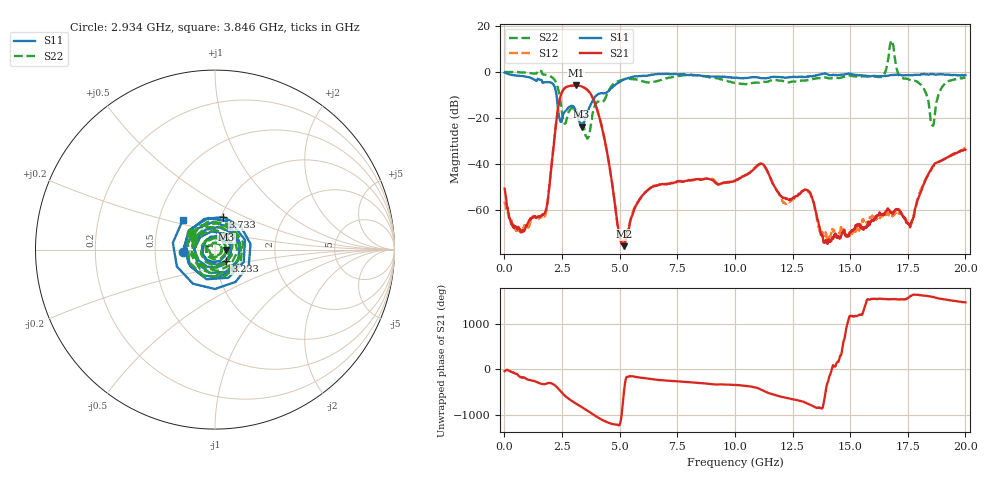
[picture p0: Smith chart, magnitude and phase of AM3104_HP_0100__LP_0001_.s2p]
!Created with skrf (http://scikit-rf.org).
# Hz S RI R 50.0
!freq ReS11 ImS11 ReS21 ImS21 ReS12 ImS12 ReS22 ImS22
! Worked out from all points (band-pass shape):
!   1601 points, 10 MHz to 20 GHz, reference 50 ohm
!   highest |S21| = -5.89 dB at 3.108 GHz (marker M1); lowest = -75.9 dB at 5.207 GHz (marker M2)
!   |S21| within 3 dB of the highest: 2.494 GHz to 3.696 GHz (1.201 GHz wide, 38.8 % of centre)
!   lowest |S11| = -23.9 dB at 3.346 GHz (marker M3), VSWR 1.14, Z = 56.8 - j0.0804 ohm
!   |S11| at or under -10 dB: 2.26 GHz to 4.026 GHz (1.766 GHz wide, 56.2 % of centre)
!   |S22| runs from -29.2 to 13.7 dB; largest |S21 - S12| = 0.028
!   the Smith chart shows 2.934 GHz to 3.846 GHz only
!   S11 on the Smith chart (normalised r, x): 2.934 GHz: 0.69, -0.02; 3.233 GHz: 1.11, -0.15; 3.733 GHz: 1.02, +0.38; 3.846 GHz: 0.66, +0.23
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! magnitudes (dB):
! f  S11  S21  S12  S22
! 10 MHz  -0.3  -50.8  -56.5  0.0
! 747.1 MHz  -1.8  -69.9  -69.1  -0.3
! 1.722 GHz  -4.6  -62.0  -62.8  -1.2
! 2.396 GHz  -20.5  -12.2  -12.2  -10.6
! 2.934 GHz  -14.8  -6.0  -6.0  -15.8
! 3.108 GHz  -17.0  -5.9  -5.9  -17.0
! 3.233 GHz  -21.2  -6.0  -6.1  -18.7
! 3.346 GHz  -23.9  -6.3  -6.4  -20.9
! 3.733 GHz  -14.6  -9.4  -9.5  -24.1
! 3.846 GHz  -12.3  -11.5  -11.5  -17.4
! 5.207 GHz  -3.2  -75.9  -74.4  -3.2
! 6.682 GHz  -0.9  -49.2  -49.3  -3.9
! 10.01 GHz  -2.6  -47.6  -47.4  -4.8
! 11.15 GHz  -2.8  -40.0  -40.2  -4.5
! 12.14 GHz  -2.5  -54.8  -56.9  -4.1
! 13.34 GHz  -2.0  -54.5  -54.7  -3.3
! 13.94 GHz  -0.8  -73.2  -70.3  -2.5
! 16.68 GHz  -1.5  -60.3  -62.5  7.2
! 17.63 GHz  -1.4  -66.7  -66.3  -3.5
! 18.56 GHz  -0.9  -41.4  -41.8  -23.3
! 19.01 GHz  -1.1  -38.4  -38.3  -6.3
! 20 GHz  -1.4  -33.9  -33.1  -2.5
